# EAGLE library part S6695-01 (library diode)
Si PIN Quadrant photodiode Source: http://sales.hamamatsu.com/assets/pdf/parts_S/S7379-01_etc.pdf
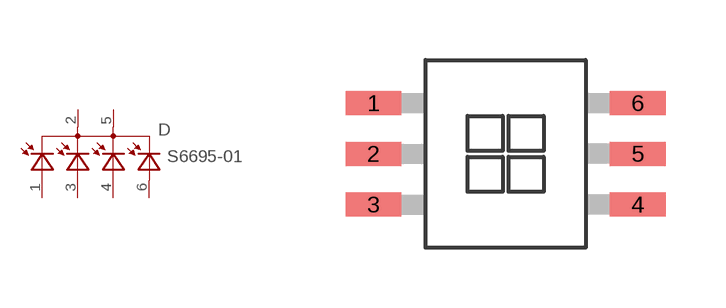
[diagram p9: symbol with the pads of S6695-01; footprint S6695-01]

Designator prefix D

## S6695-01  [S6695-01]
1  AA  pas
2  C1  pas
3  AB  pas
4  AC  pas
5  C2  pas
6  AD  pas

## Footprint S6695-01 (pad centres in mm)
Si PIN Quadrant photodiode Source: http://sales.hamamatsu.com/assets/pdf/parts_S/S7379-01_etc.pdf
smd 1.4 x 0.6: 1 -3.305,1.27; 2 -3.305,0; 3 -3.305,-1.27; 4 3.305,-1.27; 5 3.305,0; 6 3.305,1.27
